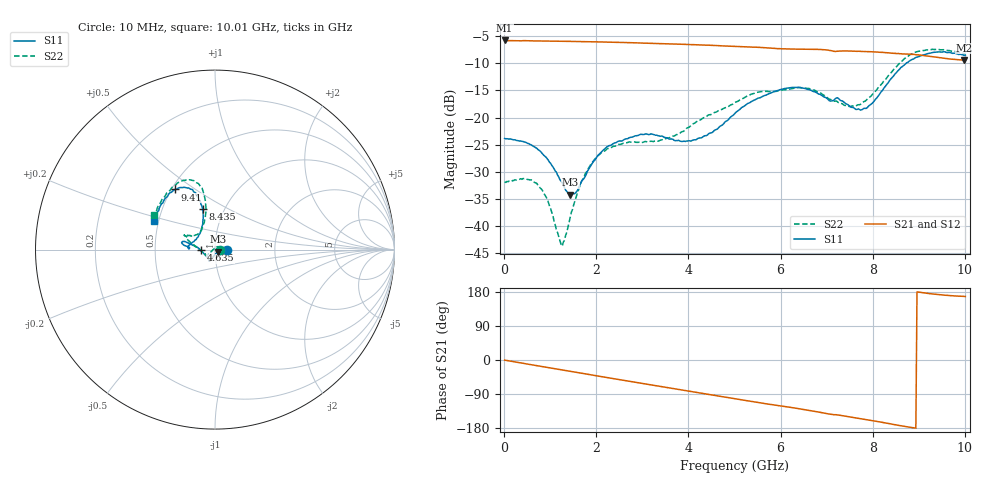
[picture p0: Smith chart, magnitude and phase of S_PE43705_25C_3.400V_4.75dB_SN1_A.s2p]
! Device ID: PE43705
! Serial: 1
! Insertion: A
! Impedance: 50 ohm
! Temp: 25C
! VDD: 3.400V
! Attenuation Step: 4.75dB
#  Hz  S  RI  R  50
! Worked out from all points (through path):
!   401 points, 10 MHz to 10.01 GHz, reference 50 ohm
!   highest |S21| = -5.80 dB at 10 MHz (marker M1); lowest = -9.4 dB at 9.985 GHz (marker M2)
!   group delay of S21, straight-line fit = 54.9 ps
!   lowest |S11| = -34.2 dB at 1.435 GHz (marker M3), VSWR 1.04, Z = 51.5 - j1.28 ohm
!   |S11| at or under -10 dB: start of sweep to 8.724 GHz
!   |S22| runs from -43.7 to -7.4 dB; largest |S21 - S12| = 0.0047
!   S11 on the Smith chart (normalised r, x): 10 MHz: 1.14, -0.00; 4.635 GHz: 0.85, -0.01; 8.435 GHz: 0.79, +0.38; 9.41 GHz: 0.52, +0.42; 10.01 GHz: 0.47, +0.17
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1e7  0.0643 -0.000213  0.513 -0.00262  0.5134 -0.00231  0.0257 8.21e-05
7.35e8  0.0493 0.0125  0.4893 -0.1351  0.4895 -0.1349  0.0157 0.0178
9.35e8  0.0409 0.00889  0.4769 -0.1701  0.4773 -0.1697  0.00922 0.0153
1.26e9  0.025 -0.00375  0.452 -0.223  0.4523 -0.2227  -0.00414 0.0051
1.435e9  0.0151 -0.0124  0.436 -0.2507  0.4363 -0.2504  -0.0121 -0.00156
1.685e9  0.00257 -0.0261  0.4101 -0.2874  0.4101 -0.2874  -0.0229 -0.0128
1.935e9  -0.00835 -0.0384  0.381 -0.3216  0.3811 -0.3213  -0.033 -0.0223
2.235e9  -0.0175 -0.0511  0.342 -0.3584  0.3423 -0.3581  -0.0417 -0.0306
3.36e9  -0.033 -0.0594  0.1709 -0.4487  0.1715 -0.4483  -0.0558 -0.025
4.01e9  -0.0504 -0.035  0.0629 -0.4662  0.0637 -0.4658  -0.0812 -0.0057
4.635e9  -0.0791 -0.00301  -0.0388 -0.4583  -0.0379 -0.4582  -0.1127 0.0215
5.01e9  -0.1082 0.0183  -0.0957 -0.4424  -0.0952 -0.4427  -0.1328 0.0371
5.985e9  -0.1748 0.0456  -0.2214 -0.3698  -0.2194 -0.3705  -0.1615 0.0731
6.685e9  -0.1741 0.0256  -0.2973 -0.3039  -0.2971 -0.3038  -0.1607 0.081
7.435e9  -0.1273 0.0394  -0.3518 -0.2124  -0.351 -0.2134  -0.0954 0.0879
7.76e9  -0.0927 0.0728  -0.37 -0.1682  -0.3693 -0.1699  -0.0731 0.1143
8.36e9  -0.0664 0.2076  -0.3856 -0.0821  -0.3849 -0.084  -0.0517 0.2447
8.435e9  -0.0691 0.2274  -0.3851 -0.0703  -0.3849 -0.0723  -0.0524 0.2664
8.86e9  -0.1193 0.3227  -0.3822 -0.0107  -0.379 -0.0134  -0.104 0.3735
9.41e9  -0.2215 0.3353  -0.3549 0.0455  -0.3537 0.0454  -0.2074 0.3725
9.985e9  -0.3327 0.1686  -0.3309 0.0717  -0.3323 0.071  -0.3301 0.2018
1.001e10  -0.3404 0.1594  -0.3319 0.0725  -0.3334 0.0718  -0.3384 0.1906
